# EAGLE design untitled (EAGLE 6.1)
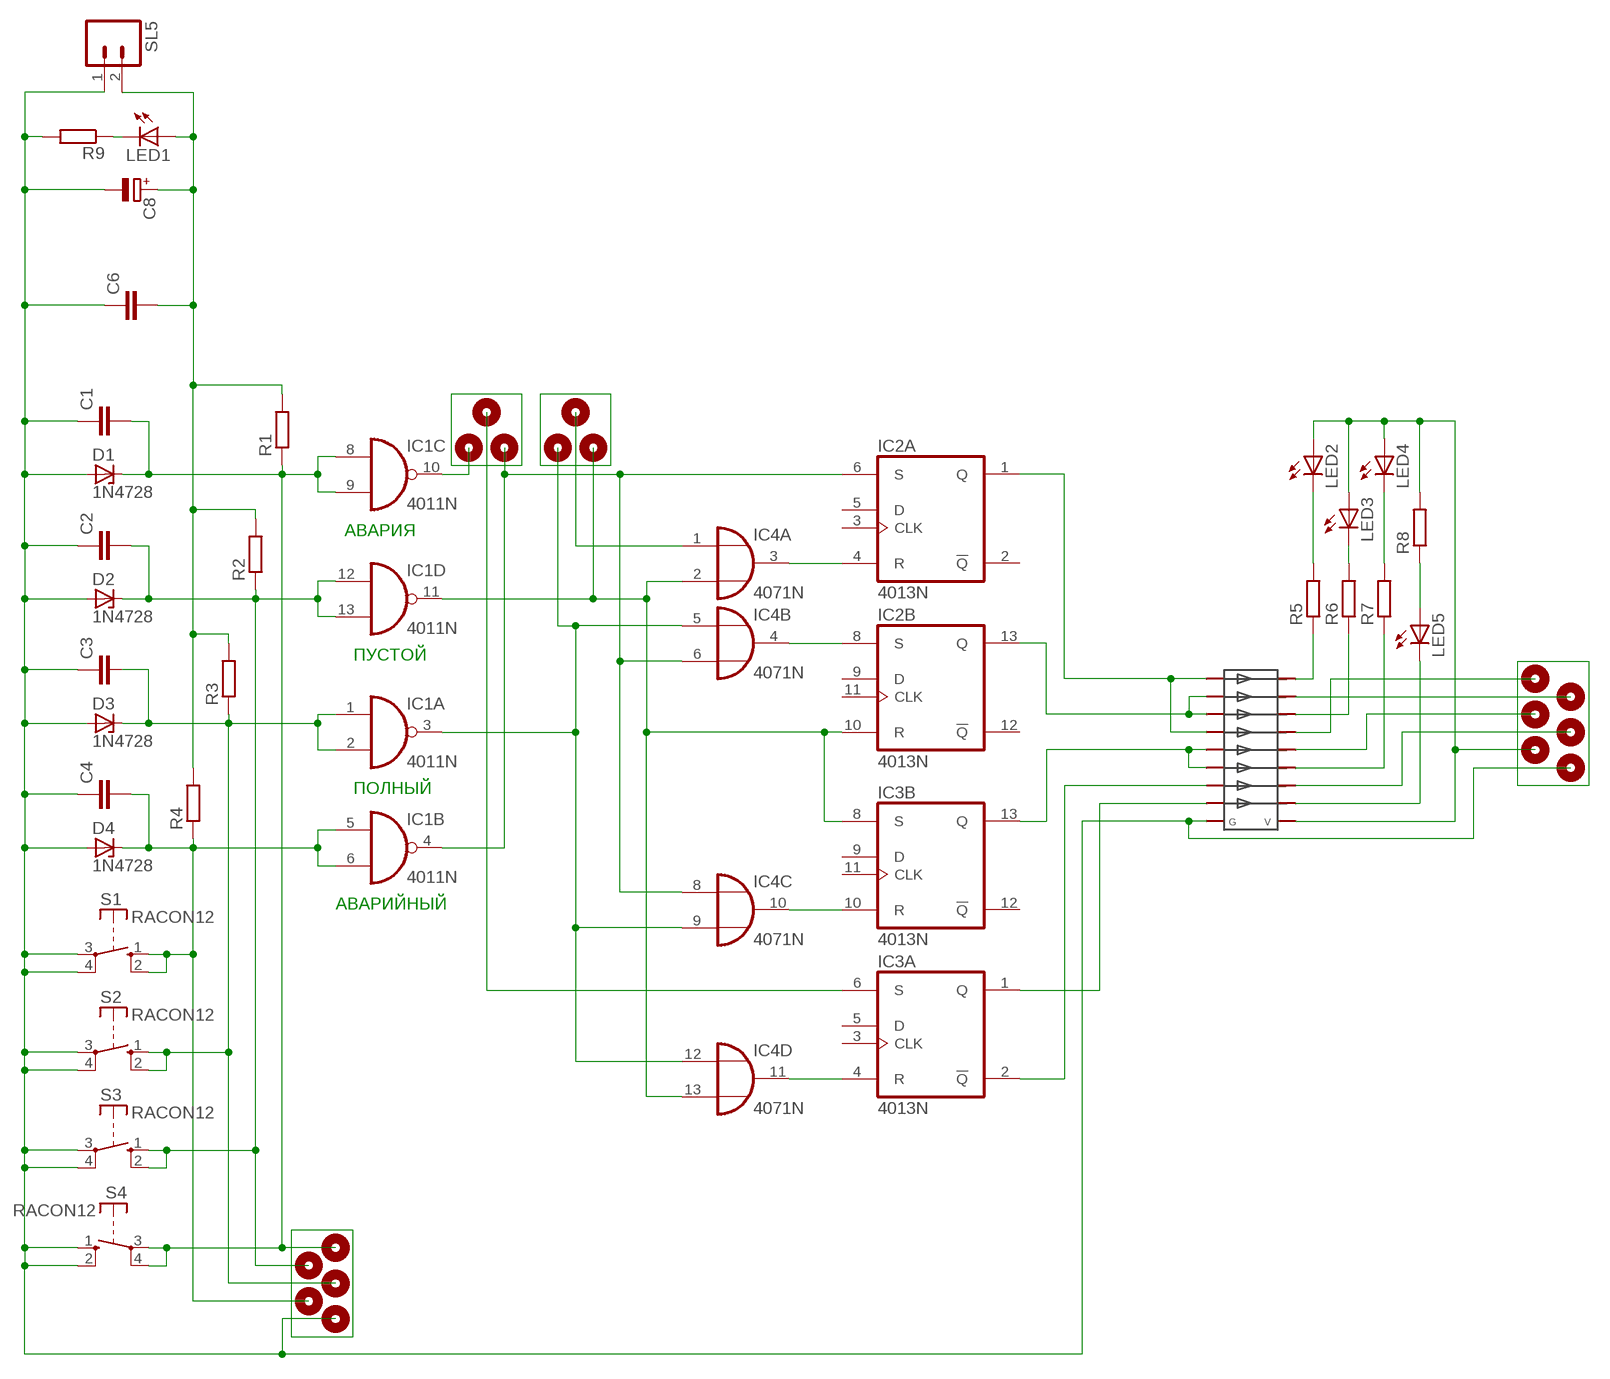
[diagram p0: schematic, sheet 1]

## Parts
C1  C-EU050-024X044  [C050-024X044]
C2  C-EU050-024X044  [C050-024X044]
C3  C-EU050-024X044  [C050-024X044]
C4  C-EU050-024X044  [C050-024X044]
C6  C-EU050-024X044  [C050-024X044]
C8  CPOL-EUE5-13  [E5-13]
D1  1N4728  [DO41Z10]
D2  1N4728  [DO41Z10]
D3  1N4728  [DO41Z10]
D4  1N4728  [DO41Z10]
IC1  4011N  [DIL14]
IC2  4013N  [DIL14]
IC3  4013N  [DIL14]
IC4  4071N  [DIL14]
IC5  2803ULN2803  [2803]
LED1  LED5MM  [LED5MM]
LED2  LED5MM  [LED5MM]
LED3  LED5MM  [LED5MM]
LED4  LED5MM  [LED5MM]
LED5  LED5MM  [LED5MM]
R1  R-EU_0207/10  [0207/10]
R2  R-EU_0207/10  [0207/10]
R3  R-EU_0207/10  [0207/10]
R4  R-EU_0207/10  [0207/10]
R5  R-EU_0207/10  [0207/10]
R6  R-EU_0207/10  [0207/10]
R7  R-EU_0207/10  [0207/10]
R8  R-EU_0207/10  [0207/10]
R9  R-EU_0207/10  [0207/10]
S1  RACON12  [RACON12]
S2  RACON12  [RACON12]
S3  RACON12  [RACON12]
S4  RACON12  [RACON12]
SL5  M02  [02P]
U$1  PIN  [PIN]
U$2  PIN  [PIN]
U$3  PIN  [PIN]
U$4  PIN  [PIN]
U$5  PIN  [PIN]
U$6  PIN  [PIN]
U$7  PIN  [PIN]
U$8  PIN  [PIN]
U$9  PIN  [PIN]
U$10  PIN  [PIN]
U$11  PIN  [PIN]
U$12  PIN  [PIN]
U$13  PIN  [PIN]
U$14  PIN  [PIN]
U$15  PIN  [PIN]
U$16  PIN  [PIN]
U$17  PIN  [PIN]

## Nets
N$1: IC5.18 R5.1
N$2: IC3.4(A:R) IC4.11(D:O)
N$3: C3.2 D3.C IC1.1(A:I0) IC1.2(A:I1) R3.1 S2.1(S) S2.2(S) U$3.1
N$4: C4.2 D4.C IC1.5(B:I0) IC1.6(B:I1) R4.1 S1.1(S) S1.2(S) U$2.1
N$5: IC5.16 R6.1
N$6: IC2.4(A:R) IC4.3(A:O)
N$7: IC1.3(A:O) IC4.5(B:I0) IC4.9(C:I1) IC4.12(D:I0) U$7.1
N$8: IC2.8(B:S) IC4.4(B:O)
N$10: IC1.11(D:O) IC2.10(B:R) IC3.8(B:S) IC4.2(A:I1) IC4.13(D:I1) U$17.1
N$11: IC3.10(B:R) IC4.10(C:O)
N$14: IC4.1(A:I0) U$6.1
N$15: IC3.6(A:S) U$9.1
N$16: IC1.4(B:O) IC2.6(A:S) IC4.6(B:I1) IC4.8(C:I0) U$8.1
N$17: IC2.1(A:Q) IC5.1 IC5.4
N$18: IC2.13(B:Q) IC5.2 IC5.3
N$19: IC3.13(B:Q) IC5.5 IC5.6
N$20: IC3.2(A:!Q) IC5.7
N$21: IC5.17 U$14.1
N$22: C1.1 C2.1 C3.1 C4.1 C6.1 C8.- D1.A D2.A D3.A D4.A IC5.9 R9.2 S1.3(P) S1.4(P) S2.3(P) S2.4(P) S3.3(P) S3.4(P) S4.1(S) S4.2(S) SL5.1 U$1.1 U$16.1
N$23: IC5.14 U$12.1
N$24: IC5.12 U$15.1
N$25: IC5.15 U$11.1
N$26: IC1.10(C:O) U$10.1
N$27: IC5.13 R7.1
N$28: IC5.11 LED5.K(C)
N$29: LED2.K(C) R5.2
N$30: LED3.K(C) R6.2
N$31: LED4.K(C) R7.2
N$32: LED5.A R8.1
N$33: IC5.10 LED2.A LED3.A LED4.A R8.2 U$13.1
N$34: LED1.K(C) R9.1
N$47: C2.2 D2.C IC1.12(D:I0) IC1.13(D:I1) R2.1 S3.1(S) S3.2(S) U$4.1
N$48: C1.2 D1.C IC1.8(C:I0) IC1.9(C:I1) R1.1 S4.3(P) S4.4(P) U$5.1
N$176: IC3.1(A:Q) IC5.8
VDD: C6.2 C8.+ LED1.A R1.2 R2.2 R3.2 R4.2 SL5.2
Unconnected: IC2.2(A:!Q) IC2.3(A:CLK) IC2.5(A:D) IC2.9(B:D) IC2.11(B:CLK) IC2.12(B:!Q) IC3.3(A:CLK) IC3.5(A:D) IC3.9(B:D) IC3.11(B:CLK) IC3.12(B:!Q)

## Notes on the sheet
- АВАРИЯ
- ПУСТОЙ
- ПОЛНЫЙ
- АВАРИЙНЫЙ

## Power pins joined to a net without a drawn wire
VDD: IC1.14(P:VDD) IC2.14(P:VDD) IC3.14(P:VDD) IC4.14(P:VDD)
VSS: IC1.7(P:VSS) IC2.7(P:VSS) IC3.7(P:VSS) IC4.7(P:VSS)

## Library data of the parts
C1-C4 C6 = rcl:C-EU: CAPACITOR, European symbol
C8 = rcl:CPOL-EU: POLARIZED CAPACITOR, European symbol
D1-D4 = diode:1N4728: Z DIODE
IC1 = 40xx:4011: Quad 2-input NAND
IC2 IC3 = 40xx:4013: Dual D FLIP FLOP, set/reset
IC4 = 40xx:4071: Quad 2-input OR
IC5 = untitled:2803
LED1-LED5 = led:LED: LED
R1-R9 = rcl:R-EU_: RESISTOR, European symbol
S1-S4 = switch-misc:RACON12: ITT SWITCH
SL5 = con-amp-quick:M02: AMP QUICK CONNECTOR; OC_FARNELL: unknown; OC_NEWARK: unknown
U$1-U$17 = untitled:PIN

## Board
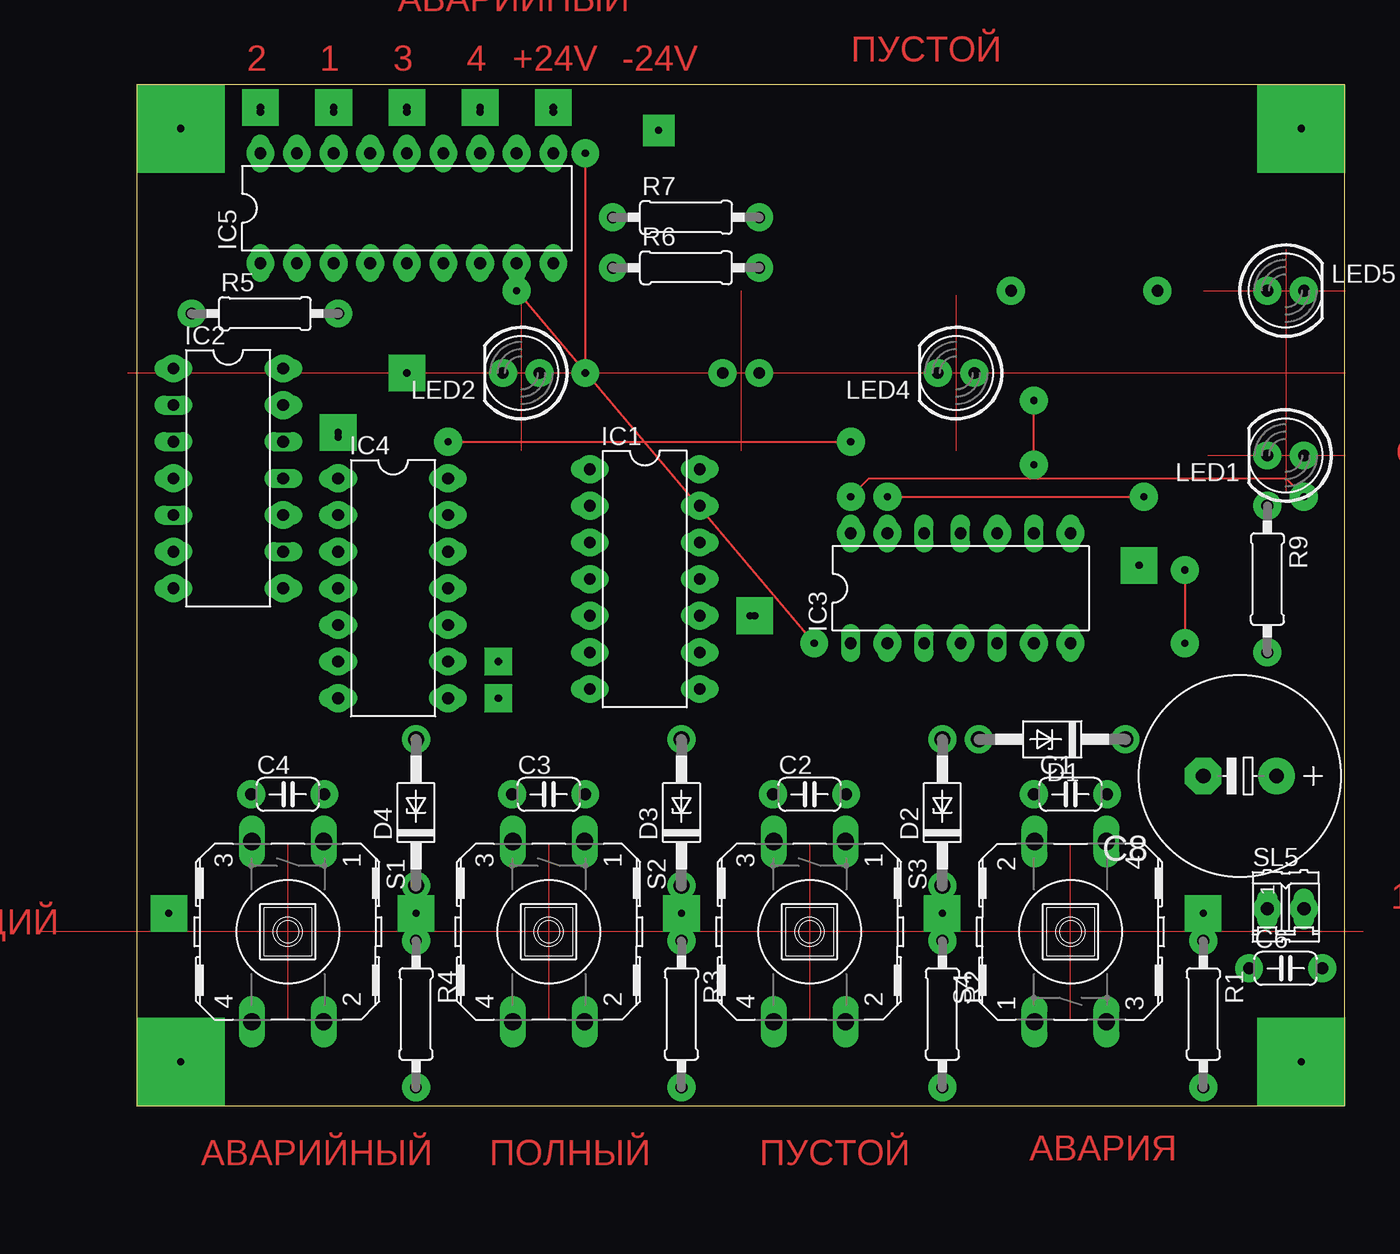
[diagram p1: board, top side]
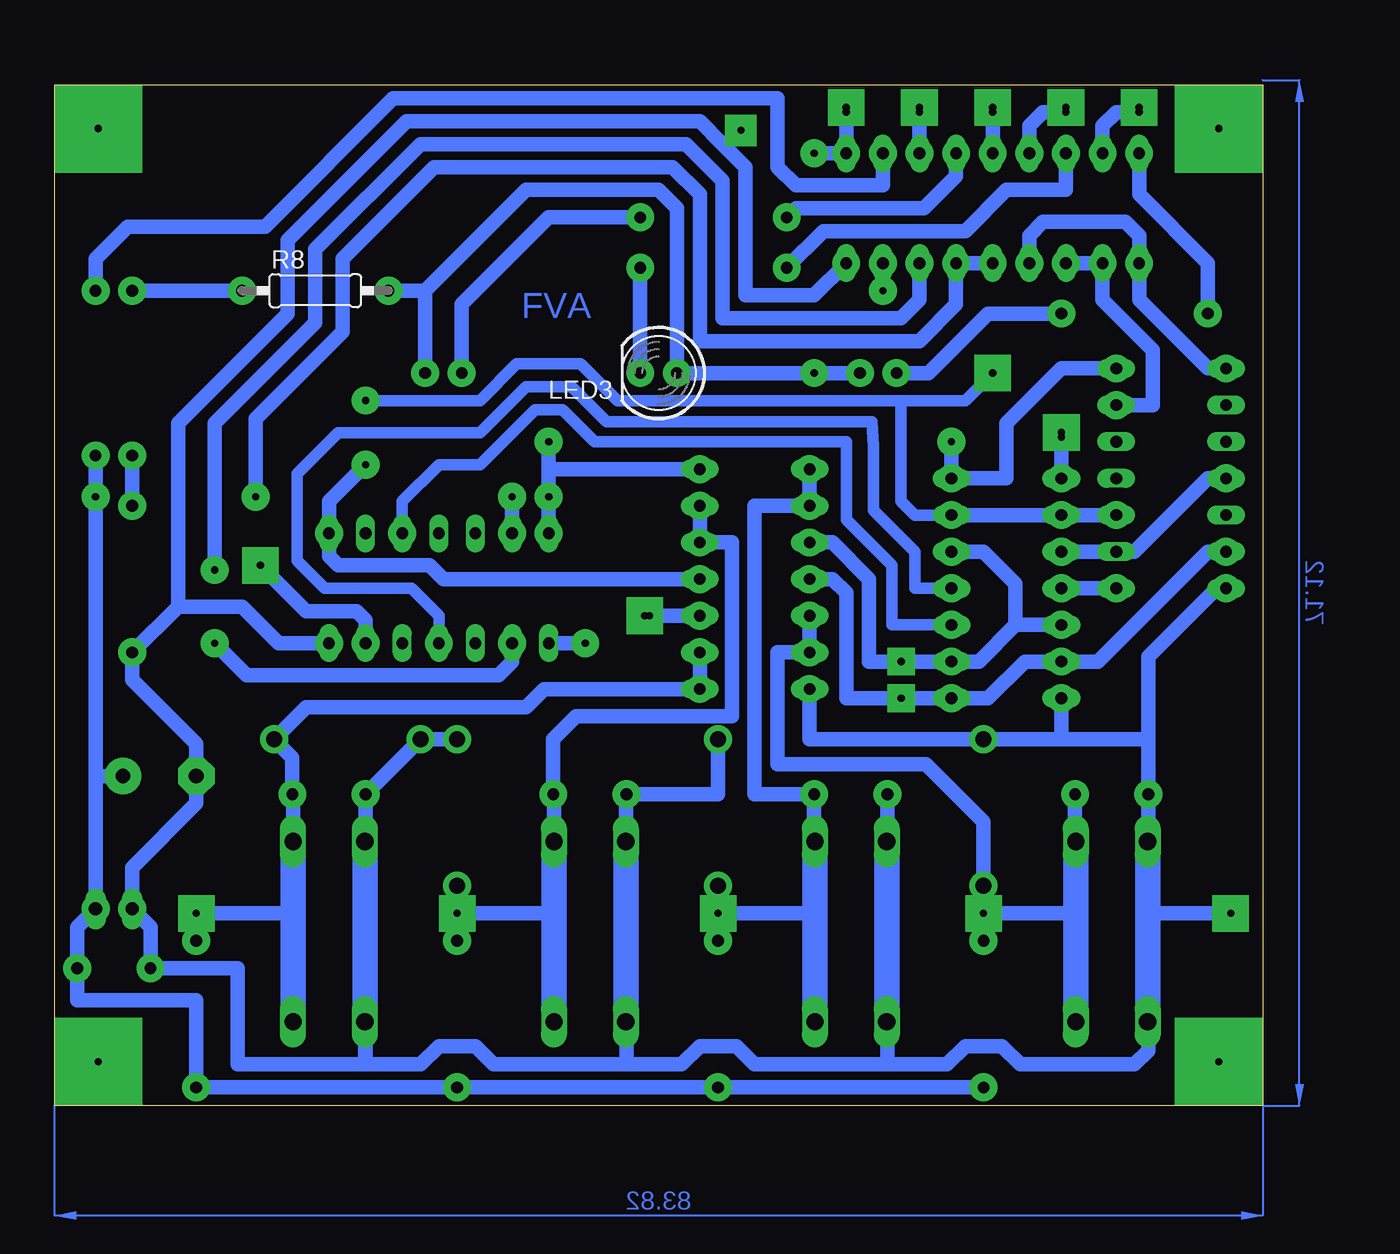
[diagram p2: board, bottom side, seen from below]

Size 83.8 x 70.79 mm. Coordinates in mm from the lower left corner, seen from the top.
Outline: 0,0 83.8,0 83.8,70.79 0,70.79 0,0
Copper layers (1*16): Top 0.035mm / dielectric 1.5mm / Bottom 0.035mm
Design rules: minimum track width 10mil, minimum drill 24mil, track to track 8mil, track to pad 8mil, pad to pad 8mil, via to via 8mil, smd to smd 8mil, copper to edge 40mil, drill to drill 8mil, minimum pad ring 10mil, minimum via ring 8mil, stop-mask expansion 4mil, vias tented up to drill 0mil, thermal gap 10mil

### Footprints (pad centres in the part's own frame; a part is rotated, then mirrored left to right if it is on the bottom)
C050-024X044 = drill 0.813 octagon: 1 -2.54,0; 2 2.54,0
E5-13 = drill 1.016 pad 2.54: + -2.54,0 | drill 1.016 pad 2.54 octagon: - 2.54,0
DO41Z10 = drill 1.118: A 5.08,0; C -5.08,0
DIL14 = drill 0.813 long: 1 -7.62,-3.81; 2 -5.08,-3.81; 3 -2.54,-3.81; 4 0,-3.81; 5 2.54,-3.81; 6 5.08,-3.81; 7 7.62,-3.81; 8 7.62,3.81; 9 5.08,3.81; 10 2.54,3.81; 11 0,3.81; 12 -2.54,3.81; 13 -5.08,3.81; 14 -7.62,3.81
2803 = drill 0.813 long: 1 -10.16,-3.81; 2 -7.62,-3.81; 3 -5.08,-3.81; 4 -2.54,-3.81; 5 0,-3.81; 6 2.54,-3.81; 7 5.08,-3.81; 8 7.62,-3.81; 9 10.16,-3.81; 10 10.16,3.81; 11 7.62,3.81; 12 5.08,3.81; 13 2.54,3.81; 14 0,3.81; 15 -2.54,3.81; 16 -5.08,3.81; 17 -7.62,3.81; 18 -10.16,3.81
LED5MM = drill 0.813 octagon: A -1.27,0; K 1.27,0
0207/10 = drill 0.813 octagon: 1 -5.08,0; 2 5.08,0
RACON12 = drill 1.194 long: 1 -6.248,2.489; 2 6.248,2.489; 3 -6.248,-2.489; 4 6.248,-2.489
02P = drill 0.914 long: 1 -1.27,0; 2 1.27,0
PIN = drill 0.5 pad 1.676 square: 1 0,0

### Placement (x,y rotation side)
C1  64.77,21.59 0 top
C2  46.67,21.59 0 top
C3  28.57,21.59 0 top
C4  10.48,21.59 0 top
C6  79.69,9.53 0 top
C8  76.52,22.86 180 top
D1  63.5,25.4 180 top
D2  55.88,20.32 90 top
D3  37.78,20.32 90 top
D4  19.37,20.32 90 top
IC1  35.24,36.51 270 top
IC2  6.35,43.5 270 top
IC3  57.15,35.88 0 top
IC4  17.78,35.88 270 top
IC5  18.73,62.23 0 top
LED1  79.69,45.09 180 top
LED2  26.67,50.8 180 top
LED3  41.91,50.8 180 bottom
LED4  56.83,50.8 180 top
LED5  79.69,56.52 0 top
R1  73.98,6.35 270 top
R2  55.88,6.35 270 top
R3  37.78,6.35 270 top
R4  19.37,6.35 270 top
R5  8.89,54.93 0 top
R6  38.1,58.1 0 top
R7  38.1,61.59 0 top
R8  65.72,56.52 0 bottom
R9  78.42,36.51 270 top
S1  10.48,12.06 270 top
S2  28.57,12.06 270 top
S3  46.67,12.06 270 top
S4  64.77,12.06 90 top
SL5  79.69,13.65 0 top
U$1  2.22,13.34 0 top
U$2  19.37,13.34 0 top
U$3  37.78,13.34 0 top
U$4  55.88,13.34 0 top
U$5  73.98,13.34 0 top
U$6  13.97,46.35 0 top
U$7  25.08,30.8 0 top
U$8  25.08,28.26 0 top
U$9  69.53,37.47 0 top
U$10  42.55,33.97 0 top
U$11  13.65,68.9 0 top
U$12  18.73,68.9 0 top
U$13  28.89,68.9 0 top
U$14  8.57,68.9 0 top
U$15  23.81,68.9 0 top
U$16  36.2,67.63 0 top
U$17  18.73,50.8 0 top

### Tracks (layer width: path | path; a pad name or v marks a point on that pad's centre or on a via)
N$1
  Bottom 1.016: R5.1 3.81,58.42 8.57,63.18 IC5.18
N$2
  Bottom 0.813: IC4.11 24.13,35.88 24.13,38.42 26.99,41.27 26.99,45.72 27.11,47.43 45.53,47.43 47.94,49.85 51.12,49.85 54.29,46.67 64.14,46.67 66.99,43.81 66.99,37.78 65.09,35.88 59.05,35.88 57.15,33.97 IC3.4
N$3
  Bottom 1.016: U$3.1 R3.1 | D3.C U$3.1 | U$3.1 31.06,13.34 | S2.1 31.11,18.31 C3.2 35.24,21.59 35.24,41.59 IC1.2 IC1.1
  Bottom 1.778: S2.1 31.06,13.34 S2.2
N$4
  Bottom 1.016: R4.1 U$2.1 | U$2.1 12.97,13.34 | C4.2 13.02,18.31 S1.1 | IC1.5 IC1.6 33.66,31.43 33.66,23.69 23.37,23.69 19.37,19.68 D4.C U$2.1
  Bottom 1.778: S1.1 12.97,13.34 S1.2
N$5
  Bottom 1.016: IC5.16 13.65,63.5 17.78,63.5 20.64,60.64 30.48,60.64 R6.1
N$6
  Bottom 1.016: IC4.3 8.89,38.42 3.81,43.5 IC2.4
N$7
  Bottom 1.016: 17.14,33.34 19.68,30.8 IC4.9 U$7.1 27.3,30.8 27.3,36.51 29.84,39.05 IC1.3 | 17.14,33.34 17.14,36.2 19.37,38.42 IC4.12 | IC4.5 17.14,33.34
N$8
  Bottom 1.016: IC2.8 IC4.4
N$10  (via drill 0.5 pad 1.93)
  Top 0.127: v62.23,44.45 v62.23,48.9
  Bottom 0.813: IC4.13 24.13,40.96 25.08,41.91 25.08,48.9 | 25.08,48.9 44.77,48.9 47.31,51.44 51.75,51.44 54.29,48.9 v62.23,48.9 | U$17.1 20.64,48.9 25.08,48.9
  Bottom 1.016: IC4.13 IC4.2 IC2.10 | IC1.11 56.83,36.51 57.78,37.47 64.14,37.47 64.77,38.1 IC3.8 64.77,41.91 v62.23,44.45
N$11
  Bottom 0.813: IC4.10 25.72,33.34 25.72,37.47 28.89,40.64 28.89,46.04 46.35,46.04 48.58,48.26 50.48,48.26 54.29,44.45 57.15,44.45 59.69,41.91 IC3.10
N$12  (via drill 0.5 pad 1.93)
  other vias: 28.89,66.04
N$13  (via drill 0.5 pad 6.1)
  other vias: 3.05,67.75
N$14
  Bottom 1.016: IC4.1 U$6.1
N$15
  Bottom 1.016: U$9.1 66.36,34.29 62.87,34.29 62.23,33.66 IC3.6
N$16
  Bottom 1.016: IC2.6 3.81,38.42 11.43,30.8 IC4.6 16.51,30.8 19.05,28.26 IC4.8 U$8.1 28.89,28.26 28.89,35.56 29.84,36.51 IC1.4
N$17
  Bottom 1.016: IC5.4 16.19,60.33 15.24,61.28 9.53,61.28 8.57,60.33 IC5.1 8.57,55.88 3.81,51.12 IC2.1
N$18
  Bottom 1.016: IC2.13 7.62,48.58 7.62,52.39 11.11,55.88 IC5.2 IC5.3
N$19  (via drill 0.5 pad 1.93)
  Top 0.127: v52.07,42.23 v69.85,42.23
  Bottom 1.016: IC5.5 IC5.6 21.27,55.56 23.81,53.02 39.05,53.02 39.05,63.18 40.96,65.09 57.47,65.09 63.82,58.74 63.82,53.66 69.85,47.62 v69.85,42.23 | IC3.13 v52.07,42.23
N$20  (via drill 0.5 pad 1.93)
  Top 0.127: v72.71,37.15 v72.71,32.07
  Bottom 1.016: IC3.2 52.07,30.8 53.02,29.84 70.48,29.84 v72.71,32.07 | v72.71,37.15 72.71,47.31 65.72,54.29 65.72,59.37 58.42,66.67 40.01,66.67 37.47,64.14 37.47,54.61 25.08,54.61 23.81,55.88 IC5.7
N$21
  Bottom 1.016: U$14.1 10.16,68.9 11.11,67.94 IC5.17
N$22
  Bottom 1.016: S3.4 44.13,5.82 44.13,2.86 | 44.13,2.86 53.34,2.86 54.61,4.13 57.15,4.13 58.42,2.86 62.23,2.86 62.23,5.77 S4.1 62.28,2.86 71.12,2.86 71.12,9.53 C6.1 77.15,12.38 SL5.1 78.42,16.51 73.98,20.95 C8.- 73.98,25.08 78.42,29.53 R9.2 75.25,34.61 75.25,47.31 67.63,54.93 67.63,60.01 59.37,68.26 39.05,68.26 37.47,66.67 | 44.13,2.86 40.32,2.86 39.05,4.13 36.51,4.13 35.24,2.86 26.04,2.86 | 26.04,2.86 26.04,5.77 S2.4 | 26.04,2.86 21.91,2.86 20.64,4.13 18.1,4.13 16.83,2.86 8.89,2.86 7.94,3.81 7.94,5.77 S1.4 | S1.3 7.94,18.31 C4.1 7.94,25.4 D4.A | S3.3 44.18,21.91 C2.1 37.78,21.59 D3.A | U$1.1 7.99,13.34 | D2.A D1.A C1.1 62.23,18.31 S4.2 | C3.1 26.04,18.31 S2.3 | IC5.9 31.11,56.2 35.88,56.2 35.88,65.09 37.47,66.67 | U$16.1 37.15,66.67 37.47,66.67
  Bottom 1.778: S1.3 7.99,13.34 S1.4 | S4.1 S4.2 | S2.3 S2.4 | S3.4 S3.3
N$23
  Bottom 1.016: IC5.14 U$12.1
N$24
  Bottom 1.016: IC5.12 U$15.1
N$25
  Bottom 1.016: IC5.15 16.19,67.94 15.24,68.9 U$11.1
N$26
  Bottom 1.016: IC1.10 U$10.1
N$27
  Bottom 1.016: IC5.13 21.27,64.45 23.5,62.23 32.38,62.23 R7.1
N$28
  Bottom 1.016: IC5.11 26.35,63.82 32.38,63.82 33.66,65.09 33.66,69.85 60.33,69.85 69.22,60.96 78.74,60.96 80.96,58.74 LED5.K
N$29
  Bottom 1.016: R5.2 19.05,54.93 23.18,50.8 LED2.K
N$30
  Bottom 1.016: LED3.K R6.2
N$31
  Bottom 1.016: R7.2 49.53,61.59 55.56,55.56 LED4.K
N$32
  Bottom 1.016: R8.1 LED5.A
N$33  (via drill 0.5 pad 1.93)
  Top 0.127: v31.11,50.8 v31.11,66.04
  Bottom 1.016: U$13.1 IC5.10 v31.11,66.04 | LED4.A 58.1,56.52 | R8.2 58.1,56.52 | 58.1,56.52 51.12,63.5 41.91,63.5 40.64,62.23 LED3.A v31.11,50.8 LED2.A
  other vias: 60.64,56.52
N$34
  Bottom 1.016: R9.1 LED1.K
N$35
  Top 0: 85.09,12.06 -6.99,12.06
N$36
  Top 0: 83.82,50.8 -0.64,50.8
N$37
  Top 0: 41.91,56.52 41.91,45.4
N$38
  Top 0: 26.67,56.52 26.67,45.4
N$39
  Top 0: 56.83,56.2 56.83,45.4
N$40
  Top 0: 79.69,59.37 79.69,42.55
N$41
  Top 0: 64.77,6.03 64.77,18.1
N$42
  Top 0: 46.67,18.1 46.67,6.03
N$43
  Top 0: 28.57,18.1 28.57,6.03
N$44
  Top 0: 10.48,18.1 10.48,6.03
N$45
  Top 0: 74.3,45.09 83.82,45.09
N$46
  Top 0: 73.98,56.52 83.82,56.52
N$47
  Bottom 1.016: U$4.1 R2.1 | D2.C U$4.1 | U$4.1 49.16,13.34 | S3.1 49.16,21.91 C2.2 49.21,25.4 47.62,26.99 36.83,26.99 36.83,39.05 IC1.12 IC1.13
  Bottom 1.778: S3.1 49.16,13.34 S3.2
N$48
  Bottom 1.016: R1.1 U$5.1 67.26,13.34 | S4.4 67.26,21.91 C1.2 67.31,24.13 D1.C 66.36,27.62 51.12,27.62 49.85,28.89 IC1.8 IC1.9
  Bottom 1.778: S4.3 67.26,13.34 S4.4
N$49  (via drill 0.5 pad 2.54)
  other vias: 2.22,13.34
N$50  (via drill 0.5 pad 2.54)
  other vias: 19.37,13.34
N$51  (via drill 0.5 pad 1.93)
  other vias: 11.11,58.42
N$52  (via drill 0.5 pad 1.93)
  other vias: 43.18,61.59
N$53  (via drill 0.5 pad 1.93)
  other vias: 33.02,61.59
N$54  (via drill 0.5 pad 1.93)
  other vias: 33.02,58.1
N$55  (via drill 0.5 pad 1.93)
  other vias: 28.89,58.42
N$56  (via drill 0.5 pad 1.93)
  other vias: 26.35,58.42
N$57  (via drill 0.5 pad 1.93)
  other vias: 23.81,58.42
N$58  (via drill 0.5 pad 1.93)
  other vias: 21.27,58.42
N$59  (via drill 0.5 pad 1.93)
  other vias: 18.73,58.42
N$60  (via drill 0.5 pad 1.93)
  other vias: 16.19,58.42
N$61  (via drill 0.5 pad 1.93)
  other vias: 13.65,58.42
N$62  (via drill 0.5 pad 1.93)
  other vias: 8.57,58.42
N$63  (via drill 0.5 pad 1.93)
  other vias: 8.57,66.04
N$64  (via drill 0.5 pad 1.93)
  other vias: 11.11,66.04
N$65  (via drill 0.5 pad 1.93)
  other vias: 13.65,66.04
N$66  (via drill 0.5 pad 1.93)
  other vias: 16.19,66.04
N$67  (via drill 0.5 pad 1.93)
  other vias: 18.73,66.04
N$68  (via drill 0.5 pad 1.93)
  other vias: 21.27,66.04
N$69  (via drill 0.5 pad 1.93)
  other vias: 23.81,66.04
N$70  (via drill 0.5 pad 1.93)
  other vias: 26.35,66.04
N$71  (via drill 0.5 pad 1.93)
  other vias: 52.07,39.69
N$72  (via drill 0.5 pad 1.93)
  other vias: 58.1,50.8
N$73  (via drill 0.5 pad 1.93)
  other vias: 55.56,50.8
N$74  (via drill 0.5 pad 1.93)
  other vias: 43.18,50.8
N$75  (via drill 0.5 pad 1.93)
  other vias: 40.64,50.8
N$76  (via drill 0.5 pad 1.93)
  other vias: 27.94,50.8
N$77  (via drill 0.5 pad 1.93)
  other vias: 25.4,50.8
N$78  (via drill 0.5 pad 1.93)
  other vias: 39.05,44.13
N$79  (via drill 0.5 pad 1.93)
  other vias: 3.81,54.93
N$80  (via drill 0.5 pad 1.93)
  other vias: 13.97,28.26
N$81  (via drill 0.5 pad 1.93)
  other vias: 13.97,30.8
N$82  (via drill 0.5 pad 1.93)
  other vias: 21.59,28.26
N$83  (via drill 0.5 pad 1.93)
  other vias: 21.59,30.8
N$84  (via drill 0.5 pad 1.93)
  other vias: 21.59,33.34
N$85  (via drill 0.5 pad 1.93)
  other vias: 13.97,33.34
N$86  (via drill 0.5 pad 1.93)
  other vias: 10.16,35.88
N$87  (via drill 0.5 pad 1.93)
  other vias: 21.59,35.88
N$88  (via drill 0.5 pad 1.93)
  other vias: 13.97,35.88
N$89  (via drill 0.5 pad 1.93)
  other vias: 13.97,38.42
N$90  (via drill 0.5 pad 1.93)
  other vias: 13.97,40.96
N$91  (via drill 0.5 pad 1.93)
  other vias: 2.54,35.88
N$92  (via drill 0.5 pad 1.93)
  other vias: 2.54,38.42
N$93  (via drill 0.5 pad 1.93)
  other vias: 21.59,38.42
N$94  (via drill 0.5 pad 1.93)
  other vias: 21.59,40.96
N$95  (via drill 0.5 pad 1.93)
  other vias: 21.59,43.5
N$96  (via drill 0.5 pad 1.93)
  other vias: 13.97,43.5
N$97  (via drill 0.5 pad 1.93)
  other vias: 2.54,43.5
N$98  (via drill 0.5 pad 1.93)
  other vias: 10.16,48.58
N$99  (via drill 0.5 pad 1.93)
  other vias: 10.16,51.12
N$100  (via drill 0.5 pad 1.93)
  other vias: 2.54,51.12
N$101  (via drill 0.5 pad 1.93)
  other vias: 10.16,40.96
N$102  (via drill 0.5 pad 1.93)
  other vias: 43.18,58.1
N$103  (via drill 0.5 pad 1.93)
  other vias: 70.8,56.52
N$104  (via drill 0.5 pad 1.93)
  other vias: 78.42,56.52
N$105  (via drill 0.5 pad 1.93)
  other vias: 13.97,54.93
N$106  (via drill 0.5 pad 1.93)
  other vias: 31.43,44.13
N$107  (via drill 0.5 pad 1.93)
  other vias: 80.96,56.52
N$108  (via drill 0.5 pad 1.93)
  other vias: 78.42,41.59
N$109  (via drill 0.5 pad 1.93)
  other vias: 78.42,31.43
N$110  (via drill 0.5 pad 1.93)
  other vias: 64.77,39.69
N$111  (via drill 0.5 pad 1.93)
  other vias: 64.77,32.07
N$112  (via drill 0.5 pad 1.93)
  other vias: 62.23,32.07
N$113  (via drill 0.5 pad 1.93)
  other vias: 57.15,32.07
N$114  (via drill 0.5 pad 1.93)
  other vias: 59.69,39.69
N$115  (via drill 0.5 pad 1.93)
  other vias: 52.07,32.07
N$116  (via drill 0.5 pad 1.93)
  other vias: 49.53,39.69
N$117  (via drill 0.5 pad 1.93)
  other vias: 78.42,45.09
N$118  (via drill 0.5 pad 1.93)
  other vias: 37.78,15.24
N$119  (via drill 0.5 pad 1.93)
  other vias: 58.42,25.4
N$120  (via drill 0.5 pad 1.93)
  other vias: 49.21,21.59
N$121  (via drill 0.5 pad 1.93)
  other vias: 44.13,21.59
N$122  (via drill 0.5 pad 1.93)
  other vias: 55.88,15.24
N$123  (via drill 0.5 pad 1.93)
  other vias: 68.58,25.4
N$124  (via drill 0.5 pad 1.93)
  other vias: 62.23,21.59
N$125  (via drill 0.5 pad 1.93)
  other vias: 55.88,25.4
N$126  (via drill 0.5 pad 1.93)
  other vias: 67.31,21.59
N$127  (via drill 0.5 pad 1.93)
  other vias: 31.43,41.59
N$128  (via drill 0.5 pad 1.93)
  other vias: 37.78,25.4
N$129  (via drill 0.5 pad 1.93)
  other vias: 39.05,28.89
N$130  (via drill 0.5 pad 1.93)
  other vias: 31.43,28.89
N$131  (via drill 0.5 pad 1.93)
  other vias: 31.43,31.43
N$132  (via drill 0.5 pad 1.93)
  other vias: 31.43,33.97
N$133  (via drill 0.5 pad 1.93)
  other vias: 39.05,31.43
N$134  (via drill 0.5 pad 1.93)
  other vias: 39.05,33.97
N$135  (via drill 0.5 pad 1.93)
  other vias: 39.05,36.51
N$136  (via drill 0.5 pad 1.93)
  other vias: 31.43,36.51
N$137  (via drill 0.5 pad 1.93)
  other vias: 31.43,39.05
N$138  (via drill 0.5 pad 1.93)
  other vias: 39.05,39.05
N$139  (via drill 0.5 pad 1.93)
  other vias: 39.05,41.59
N$140  (via drill 0.5 pad 1.93)
  other vias: 37.78,1.27
N$141  (via drill 0.5 pad 1.93)
  other vias: 19.37,11.43
N$142  (via drill 0.5 pad 1.93)
  other vias: 55.88,1.27
N$143  (via drill 0.5 pad 1.93)
  other vias: 73.98,1.27
N$144  (via drill 0.5 pad 1.93)
  other vias: 80.96,13.65
N$145  (via drill 0.5 pad 1.93)
  other vias: 73.98,11.43
N$146  (via drill 0.5 pad 1.93)
  other vias: 77.15,9.53
N$147  (via drill 0.5 pad 1.93)
  other vias: 82.23,9.53
N$148  (via drill 0.5 pad 1.93)
  other vias: 78.42,13.65
N$149  (via drill 0.5 pad 1.93)
  other vias: 31.11,21.59
N$150  (via drill 0.5 pad 1.93)
  other vias: 13.02,21.59
N$151  (via drill 0.5 pad 1.93)
  other vias: 7.94,21.59
N$152  (via drill 0.5 pad 1.93)
  other vias: 19.37,15.24
N$153  (via drill 0.5 pad 1.93)
  other vias: 37.78,11.43
N$154  (via drill 0.5 pad 1.93)
  other vias: 19.37,1.27
N$155  (via drill 0.5 pad 1.93)
  other vias: 80.96,45.09
N$156  (via drill 0.5 pad 2.54)
  other vias: 37.78,13.34
N$157  (via drill 0.5 pad 2.54)
  other vias: 55.88,13.34
N$158  (via drill 0.5 pad 2.54)
  other vias: 73.98,13.34
N$159  (via drill 0.5 pad 2.54)
  other vias: 42.86,33.97
N$160  (via drill 0.5 pad 2.54)
  other vias: 69.53,37.47
N$161  (via drill 0.5 pad 1.93)
  other vias: 25.08,28.26
N$162  (via drill 0.5 pad 1.93)
  other vias: 25.08,30.8
N$163  (via drill 0.5 pad 2.54)
  other vias: 13.97,46.67 18.73,50.8
N$164  (via drill 0.5 pad 2.54)
  other vias: 8.57,69.22
N$165  (via drill 0.5 pad 2.54)
  other vias: 13.65,69.22
N$166  (via drill 0.5 pad 2.54)
  other vias: 18.73,69.22
N$167  (via drill 0.5 pad 2.54)
  other vias: 23.81,69.22
N$168  (via drill 0.5 pad 2.54)
  other vias: 28.89,69.22
N$169  (via drill 0.5 pad 2.18)
  other vias: 36.2,67.63
N$170  (via drill 0.5 pad 1.93)
  other vias: 55.88,11.43
N$171  (via drill 0.5 pad 1.93)
  other vias: 19.37,25.4
N$172  (via drill 0.5 pad 1.93)
  other vias: 26.04,21.59
N$173  (via drill 0.5 pad 6.1)
  other vias: 80.77,67.75
N$174  (via drill 0.5 pad 6.1)
  other vias: 80.77,3.05
N$175  (via drill 0.5 pad 6.1)
  other vias: 3.05,3.05
N$176  (via drill 0.5 pad 1.93)
  Top 0.127: v26.35,56.52 v46.99,32.07
  Bottom 1.016: IC5.8 v26.35,56.52 | v46.99,32.07 IC3.1
VDD  (via drill 0.5 pad 1.93)
  Top 0.127: v21.59,46.04 v49.53,46.04 | v49.53,42.23 50.8,43.5 79.69,43.5 v80.96,42.23
  Bottom 1.016: IC2.14 13.97,51.12 17.78,47.31 17.78,43.5 IC4.14 v21.59,46.04 | IC1.14 49.53,44.13 | 49.53,44.13 v49.53,42.23 IC3.14 | v49.53,46.04 49.53,44.13 | R4.2 R3.2 R2.2 R1.2 73.98,7.3 82.23,7.3 C6.2 82.23,12.38 SL5.2 80.96,22.86 | 80.96,22.86 C8.+ | LED1.A v80.96,42.23 80.96,22.86
VSS
  Bottom 1.016: IC2.7 3.17,35.88 7.94,31.11 7.94,25.4 | 13.97,25.4 IC4.7 | IC1.7 31.43,25.4 13.97,25.4 | 13.97,25.4 7.94,25.4 | IC3.7 68.26,32.07 70.8,34.61 75.25,34.61 78.42,31.43 78.42,29.53 73.98,25.08 73.98,20.95 78.42,16.51 78.42,13.65 77.15,12.38 77.15,9.53 71.12,9.53 71.12,2.86 58.42,2.86 57.15,4.13 54.61,4.13 53.34,2.86 40.32,2.86 39.05,4.13 36.51,4.13 35.24,2.86 21.91,2.86 20.64,4.13 18.1,4.13 16.83,2.86 8.89,2.86 7.94,3.81 7.94,25.4
(copper drawn outside any net)
  shapes: Bottom area x6

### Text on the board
Top: ПОЛНЫЙ | АВАРИЙНЫЙ | 2 | 1 | 3 | 4 | +24V | -24V | ПУСТОЙ | АВАРИЯ | СЕТЬ | ОБЩИЙ | 12V | АВАРИЙНЫЙ | ПОЛНЫЙ | ПУСТОЙ | АВАРИЯ
Bottom: FVA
